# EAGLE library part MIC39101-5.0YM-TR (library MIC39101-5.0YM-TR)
LDO Voltage Regulators 1.0A 1.0% Fixed Voltage LDO Source: Datasheet
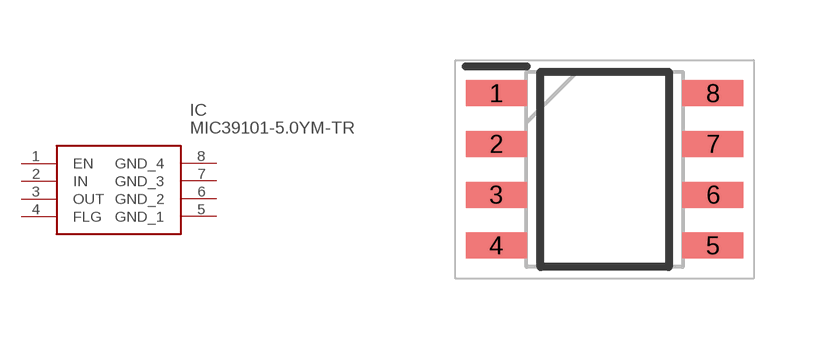
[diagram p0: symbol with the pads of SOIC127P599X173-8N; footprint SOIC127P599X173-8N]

Designator prefix IC

## MIC39101-5.0YM-TR (Description: LDO Voltage Regulators 1.0A 1.0% Fixed Voltage LDO; Height: 1.73mm; Manufacturer_Name: Microchip; Manufacturer_Part_Number: MIC39101-5.0YM-TR; Mouser_Part_Number: 998-MIC39101-5.0YMTR; Mouser_Price-Stock: https://www.mouser.co.uk/ProductDetail/Microchip-Technology-Micrel/MIC39101-50YM-TR?qs=U6T8BxXiZAW4%252Bcnkgk10yA%3D%3D)  [SOIC127P599X173-8N]
1  EN
2  IN
3  OUT
4  FLG
5  GND_1
6  GND_2
7  GND_3
8  GND_4

## Footprint SOIC127P599X173-8N (pad centres in mm)
MIC39101-5.0YM-TR
smd 1.525 x 0.65: 1 -2.712,1.905; 2 -2.712,0.635; 3 -2.712,-0.635; 4 -2.712,-1.905; 5 2.712,-1.905; 6 2.712,-0.635; 7 2.712,0.635; 8 2.712,1.905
